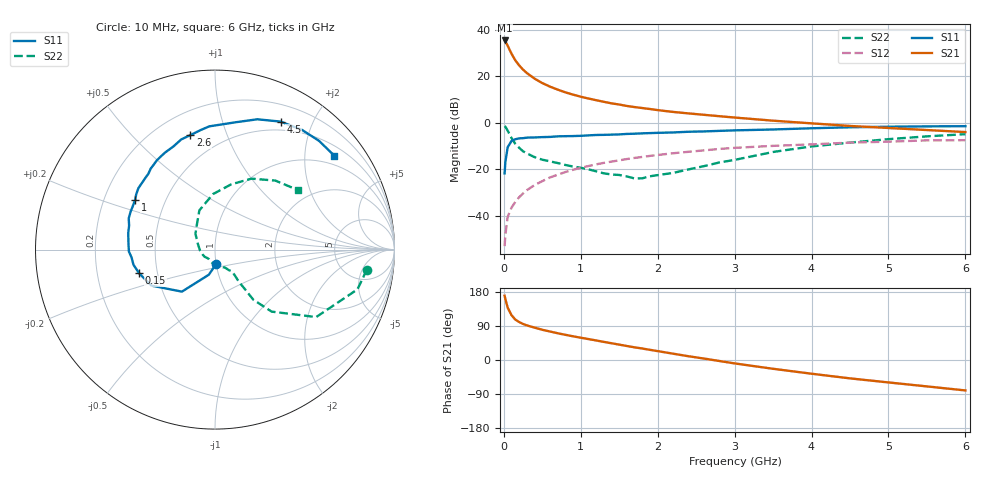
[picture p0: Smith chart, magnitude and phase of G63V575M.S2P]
! SIEMENS Small Signal Semiconductors
! BFG193
! Si NPN RF Bipolar Junction Transistor in SOT223
! VCE = 3.5 V  IC = 75 mA
! Common Emitter S-Parameters:  August  1996
# GHz  S  MA  R  50
!  f  S11  S21  S12  S22
! GHz  MAG  ANG  MAG  ANG  MAG  ANG  MAG  ANG
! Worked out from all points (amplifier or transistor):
!   36 points, 10 MHz to 6 GHz, reference 50 ohm
!   highest |S21| = 35.5 dB at 10 MHz (marker M1)
!   |S21| within 3 dB of that: start of sweep to 60.44 MHz
!   unconditionally stable (mu >= 1): start of sweep to 10.55 MHz; 298.5 MHz to 2.385 GHz
!   at 250 MHz: K = 0.99, MSG = 26.7 dB, |S12| = -30.4 dB
!   at 1.4 GHz: K = 1.06, MAG = 11.0 dB, |S12| = -16.7 dB
!   at 6 GHz: K = 0.92, MSG = 1.7 dB, |S12| = -7.5 dB
!   S11 on the Smith chart (normalised r, x): 10 MHz: 1.00, -0.16; 150 MHz: 0.39, -0.13; 1 GHz: 0.33, +0.26; 2.6 GHz: 0.34, +0.75; 4.5 GHz: 0.39, +1.56; 6 GHz: 0.73, +2.70
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0.01  0.0811 -85.8  59.5 169.8  0.0022 80.1  0.8536 -7.5
0.02  0.1441 -103.8  56.78 160.7  0.0039 77.5  0.824 -15.6
0.05  0.298 -128.2  45.76 138.1  0.0094 69.9  0.6776 -33.7
0.1  0.4073 -150.5  30.78 118.1  0.0149 66.3  0.4678 -47.6
0.15  0.4427 -162.6  22.07 106.5  0.0199 68.8  0.3517 -52.6
0.2  0.4621 -169.5  17.22 100.1  0.025 71.0  0.2891 -52.8
0.25  0.467 -174.7  13.97 95.1  0.0301 70.6  0.2435 -53.2
0.3  0.4799 -178.7  11.79 91.3  0.0354 71.6  0.2192 -53.4
0.4  0.4843 175.0  8.945 85.4  0.0456 71.2  0.1819 -52.5
0.5  0.492 169.2  7.181 79.8  0.0554 70.3  0.1606 -52.1
0.6  0.4969 164.4  6.024 75.1  0.0665 69.0  0.1479 -53.6
0.7  0.5112 160.1  5.186 70.6  0.0762 67.4  0.136 -56.4
0.8  0.5154 155.9  4.533 66.5  0.087 65.4  0.1236 -58.7
1  0.5247 147.9  3.654 58.8  0.1075 61.9  0.1076 -65.8
1.1  0.5364 144.9  3.334 55.2  0.1171 59.9  0.0996 -72.4
1.6  0.5763 128.4  2.308 36.9  0.1659 48.8  0.0699 -111.1
2.2  0.6198 111.9  1.717 16.7  0.2209 35.1  0.0833 -175.9
2.6  0.6523 102.2  1.489 3.9  0.2549 26.1  0.1164 150.6
3.5  0.7187 80.8  1.112 -23.2  0.3187 3.2  0.2355 111.7
4.5  0.8012 62.9  0.856 -48.5  0.3744 -17.1  0.375 76.0
5.5  0.8385 46.3  0.699 -69.7  0.4186 -40.7  0.5109 48.8
6  0.8458 38.3  0.632 -80.3  0.4226 -54.2  0.5693 35.6
